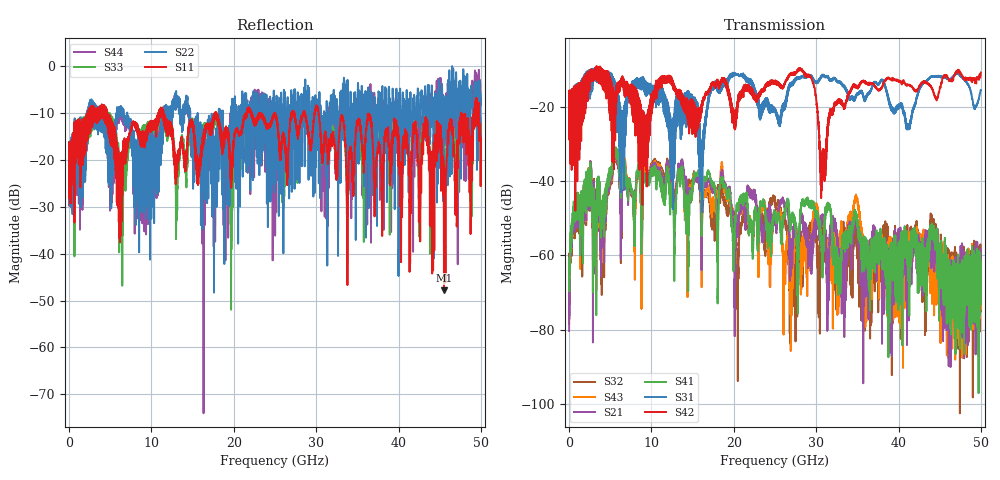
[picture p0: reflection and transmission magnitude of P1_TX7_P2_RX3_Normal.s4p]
!Keysight Technologies,N5225B,MY57041031,A.13.20.10
!Date: Friday, May 31, 2019 11:32:09
!Correction: S11(Full 4 Port(1,2,3,4))
!S12(Full 4 Port(1,2,3,4))
!S13(Full 4 Port(1,2,3,4))
!S14(Full 4 Port(1,2,3,4))
!S21(Full 4 Port(1,2,3,4))
!S22(Full 4 Port(1,2,3,4))
!S23(Full 4 Port(1,2,3,4))
!S24(Full 4 Port(1,2,3,4))
!S31(Full 4 Port(1,2,3,4))
!S32(Full 4 Port(1,2,3,4))
!S33(Full 4 Port(1,2,3,4))
!S34(Full 4 Port(1,2,3,4))
!S41(Full 4 Port(1,2,3,4))
!S42(Full 4 Port(1,2,3,4))
!S43(Full 4 Port(1,2,3,4))
!S44(Full 4 Port(1,2,3,4))
!S4P File: Measurements: <S11,S12,S13,S14>,
!<S21,S22,S23,S24>,
!<S31,S32,S33,S34>,
!<S41,S42,S43,S44>:
# Hz S  dB  R 50.0
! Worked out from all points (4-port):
!   5000 points, 10 MHz to 50 GHz, reference 50 ohm
!   strongest paths, dB at 10 MHz, 12.51 GHz, 25.01 GHz, 37.51 GHz, 50 GHz:
!     S42: -19.4, -14.3, -13.2, -15.5, -10.8
!     S31: -19.5, -38.8, -20.9, -14.0, -15.5
!     S41: -60.8, -41.0, -48.7, -58.8, -72.5
!     S21: -80.3, -39.1, -50.3, -58.5, -64.3
!     S43: -78.4, -39.2, -49.5, -63.7, -62.9
!     S32: -68.4, -37.5, -44.9, -58.6, -75.0
!   lowest |S11| = -47.8 dB at 45.52 GHz (marker M1), VSWR 1.01, Z = 49.7 + j0.256 ohm
!   |S11| at or under -10 dB: 4.613 GHz to 10.86 GHz (6.246 GHz wide, 80.7 % of centre); 11.46 GHz to 17.73 GHz (6.278 GHz wide, 43 % of centre); 30.28 GHz to 47.61 GHz (17.33 GHz wide, 44.5 % of centre)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
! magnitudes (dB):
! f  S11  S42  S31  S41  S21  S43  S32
! 10 MHz  -19.1  -19.4  -19.5  -60.8  -80.3  -78.4  -68.4
! 5.73 GHz  -15.7  -15.1  -15.2  -31.7  -32.0  -32.3  -32.6
! 16.1 GHz  -18.0  -21.2  -35.1  -52.6  -60.9  -68.6  -51.2
! 28.08 GHz  -12.0  -9.8  -12.2  -48.9  -49.8  -58.6  -55.1
! 30.78 GHz  -17.8  -33.4  -11.8  -59.2  -48.9  -50.8  -52.0
! 45.52 GHz  -47.8  -11.5  -11.9  -63.6  -64.8  -61.9  -59.6
! 50 GHz  -15.4  -10.8  -15.5  -72.5  -64.3  -62.9  -75.0
